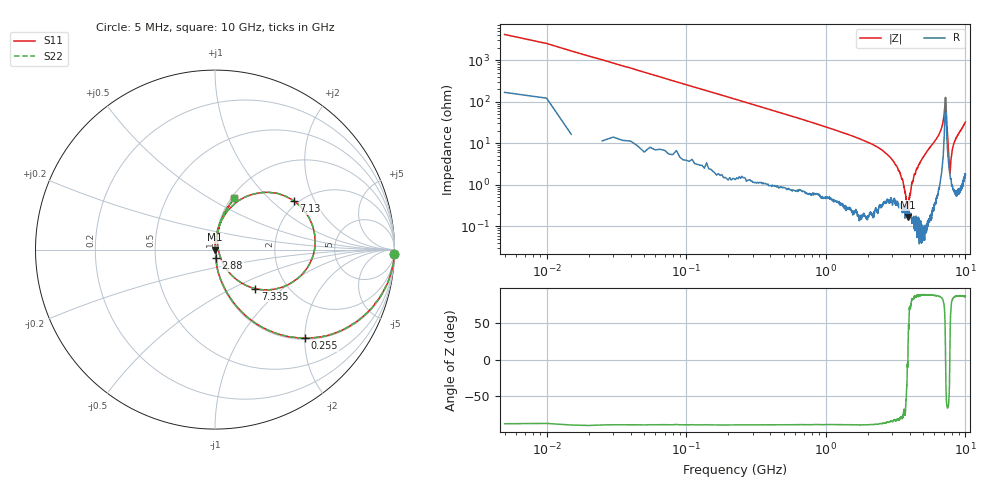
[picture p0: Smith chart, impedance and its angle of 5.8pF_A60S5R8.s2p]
! Amotech Co.,Ltd.
! http://www.amotech.co.kr/
! Part Number: A60S5R8
! These Parameters are Measured in Series Mode Connection
! Operation Temp=25[degC], DC Bias Voltage=0[V]
! Freq. Start=5[MHz] Stop=10[GHz], 2000[Steps]
! Date: Monday, July 13, 2020, 01:30:51
# GHZ S RI R 50.000000
!Freq.(Hz) S11(Real) S11(Imag) S21(Real) S21(Imag) S12(Real) S12(Imag) S22(Real) S22(Imag)
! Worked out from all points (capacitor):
!   2000 points, 5 MHz to 10 GHz, reference 50 ohm
!   read as one part in series: C = 6.23 pF near 55 MHz
!   lowest |Z| = 168 mohm at 3.875 GHz (marker M1)
!   series resonance near 3.874 GHz, so ESL is about 270 pH
!   S11 on the Smith chart (normalised r, x): 5 MHz: 4, -83; 255 MHz: 1.03, -2.01; 2.88 GHz: 1.01, -0.09; 7.13 GHz: 1.89, +1.39; 7.335 GHz: 1.39, -0.67; 10 GHz: 1.03, +0.65
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0.005  0.9984 -0.0241  0.00156 0.0241  0.00156 0.0241  0.9984 -0.0241
0.095  0.8746 -0.3238  0.1254 0.3238  0.1254 0.3238  0.8746 -0.3238
0.255  0.503 -0.4927  0.497 0.4927  0.497 0.4927  0.503 -0.4927
0.67  0.1297 -0.3267  0.8703 0.3267  0.8703 0.3267  0.1297 -0.3267
1.675  0.02 -0.132  0.98 0.132  0.98 0.132  0.02 -0.132
2.88  0.00606 -0.0459  0.9939 0.0459  0.9939 0.0459  0.00606 -0.0459
3.34  0.00368 -0.0209  0.9963 0.0209  0.9963 0.0209  0.00368 -0.0209
3.585  0.00232 -0.011  0.9977 0.011  0.9977 0.011  0.00232 -0.011
3.875  0.00167 0.000119  0.9983 -0.000119  0.9983 -0.000119  0.00167 0.000119
4.105  0.00168 0.00918  0.9983 -0.00918  0.9983 -0.00918  0.00168 0.00918
4.295  0.00126 0.017  0.9987 -0.017  0.9987 -0.017  0.00126 0.017
5.005  0.00269 0.0471  0.9973 -0.0471  0.9973 -0.0471  0.00269 0.0471
6.67  0.0528 0.1911  0.9472 -0.1911  0.9472 -0.1911  0.0528 0.1911
6.96  0.1546 0.2856  0.8454 -0.2856  0.8454 -0.2856  0.1546 0.2856
7.13  0.4383 0.2711  0.5617 -0.2711  0.5617 -0.2711  0.4383 0.2711
7.215  0.5487 -0.0254  0.4513 0.0254  0.4513 0.0254  0.5487 -0.0254
7.335  0.2255 -0.2177  0.7745 0.2177  0.7745 0.2177  0.2255 -0.2177
7.47  0.0696 -0.1162  0.9304 0.1162  0.9304 0.1162  0.0696 -0.1162
7.74  0.0182 0.00244  0.9818 -0.00244  0.9818 -0.00244  0.0182 0.00244
7.985  0.0126 0.0553  0.9874 -0.0553  0.9874 -0.0553  0.0126 0.0553
8.335  0.0174 0.1031  0.9826 -0.1031  0.9826 -0.1031  0.0174 0.1031
10  0.1079 0.2851  0.8921 -0.2851  0.8921 -0.2851  0.1079 0.2851
